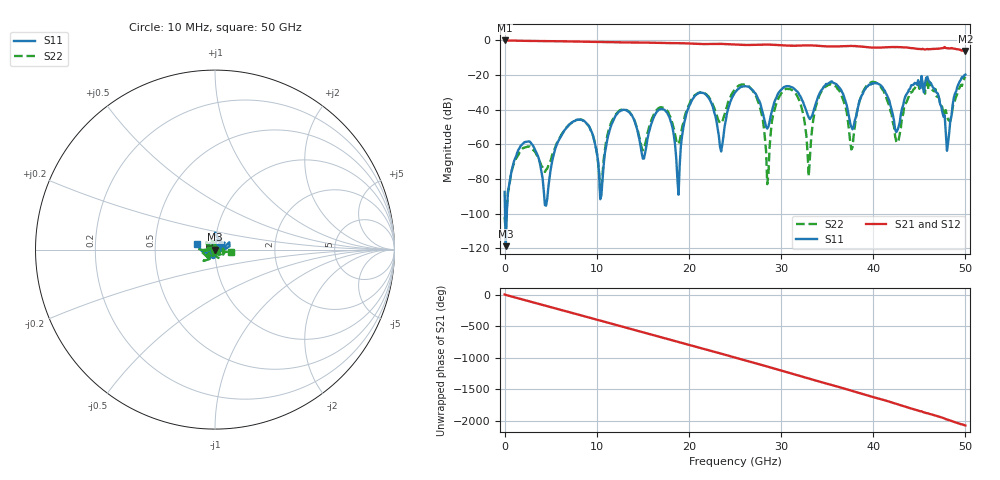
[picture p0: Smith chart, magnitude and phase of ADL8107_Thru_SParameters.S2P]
! Analog Devices, Inc.
! Device:	ADL8107ACPZN - THRU
! Description:	"GaAs, pHEMT, MMIC, Low Phase Noise Amplifier, 6 GHz to 18 GHz"
! Conditions:	Pin = -20 dBm
!		Operating Temperature = +25 C (at package bottom)
! Measurement used thru-cal line of SN#9.
! Frequency (GHz)	S11_Mag (dB)	S11_Phase (deg)	S21_Mag (dB)	S21_Phase (deg)	S12_Mag (dB)	S12_Phase (deg)	S22_Mag (dB)	S22_Phase (deg)
#  GHZ  S  DB  R 50
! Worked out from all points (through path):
!   400 points, 10 MHz to 50 GHz, reference 50 ohm
!   highest |S21| = 0.00 dB at 10 MHz (marker M1); lowest = -6.0 dB at 50 GHz (marker M2)
!   group delay of S21, straight-line fit = 114 ps
!   lowest |S11| = -118.7 dB at 135 MHz (marker M3), VSWR 1.00, Z = 50 - j0.000109 ohm
!   |S11| at or under -10 dB: start of sweep to end of sweep
!   |S22| runs from -110.2 to -20.9 dB; largest |S21 - S12| = 0.01
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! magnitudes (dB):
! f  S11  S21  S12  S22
! 10 MHz  -87.4  0.0  0.1  -101.8
! 135 MHz  -118.7  0.0  0.0  -110.2
! 8.383 GHz  -45.9  -0.7  -0.7  -45.8
! 10.51 GHz  -89.5  -0.8  -0.8  -85.8
! 12.01 GHz  -43.8  -1.0  -1.0  -43.1
! 15.13 GHz  -68.2  -1.2  -1.2  -62.7
! 16.76 GHz  -39.9  -1.5  -1.5  -38.9
! 18.88 GHz  -89.0  -1.5  -1.5  -59.4
! 20.38 GHz  -34.1  -1.9  -1.9  -33.4
! 23.51 GHz  -64.1  -2.0  -2.0  -47.8
! 25.01 GHz  -30.0  -2.4  -2.4  -28.1
! 27.5 GHz  -33.7  -2.5  -2.5  -35.2
! 28.5 GHz  -50.9  -2.4  -2.4  -83.0
! 30.13 GHz  -27.9  -2.8  -2.8  -29.6
! 32.13 GHz  -32.5  -2.9  -2.9  -36.8
! 33 GHz  -44.3  -2.8  -2.8  -78.2
! 33.38 GHz  -43.3  -2.9  -2.9  -50.7
! 41.75 GHz  -34.9  -3.9  -3.9  -37.7
! 42.63 GHz  -51.9  -3.8  -3.8  -59.0
! 45.88 GHz  -21.0  -4.9  -4.9  -24.5
! 48 GHz  -63.7  -4.5  -4.5  -43.7
! 50 GHz  -19.7  -6.0  -5.9  -21.0
